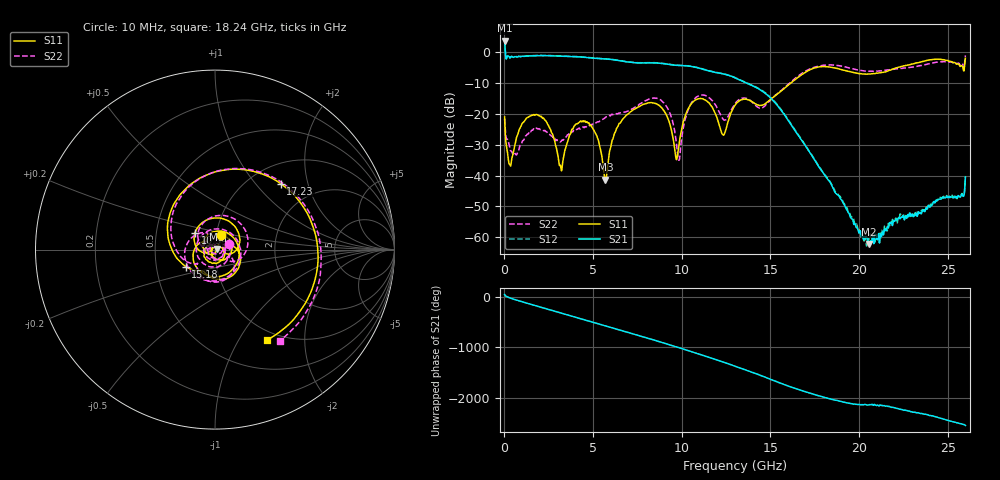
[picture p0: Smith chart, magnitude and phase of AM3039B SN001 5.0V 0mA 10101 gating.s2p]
!Agilent Technologies,E8364B,MY43040894,A.07.50.67
!Agilent E8364B: A.07.50.67
!Date: Tuesday, June 28, 2016 08:09:14
!Correction: S11(Full 2 Port(1,2))
!S21(Full 2 Port(1,2))
!S12(Full 2 Port(1,2))
!S22(Full 2 Port(1,2))
!S2P File: Measurements: S11, S21, S12, S22:
# Hz S  dB  R 50
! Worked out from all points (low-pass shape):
!   1601 points, 10 MHz to 26 GHz, reference 50 ohm
!   highest |S21| = 3.74 dB at 10 MHz (marker M1); lowest = -62.1 dB at 20.57 GHz (marker M2)
!   |S21| within 3 dB of the highest: start of sweep to 44.01 MHz
!   lowest |S11| = -41.3 dB at 5.695 GHz (marker M3), VSWR 1.02, Z = 50.9 + j0.0578 ohm
!   |S11| at or under -10 dB: start of sweep to 16.15 GHz
!   |S22| runs from -35.0 to -1.1 dB; largest |S21 - S12| = 0.025
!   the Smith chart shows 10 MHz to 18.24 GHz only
!   S11 on the Smith chart (normalised r, x): 10 MHz: 1.05, +0.18; 10.54 GHz: 0.79, +0.15; 15.18 GHz: 0.71, -0.14; 17.23 GHz: 1.36, +1.37; 18.24 GHz: 0.87, -1.33
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1e7  -20.97 68.1  3.74 40.9  3.81 41.8  -21.66 20.3
7.409688e8  -26.77 125.0  -1.51 -74.4  -1.46 -74.2  -32.56 179.9
1.69935e9  -20.40 28.8  -1.14 -172.8  -1.11 -172.6  -24.74 16.6
2.755194e9  -27.28 -101.1  -1.19 81.3  -1.12 81.5  -27.99 -159.7
3.551138e9  -29.23 21.2  -1.35 1.9  -1.28 2.0  -26.81 27.3
4.347081e9  -22.47 -91.2  -1.57 -78.8  -1.53 -78.7  -24.45 -116.6
5.695312e9  -41.34 3.8  -2.20 144.2  -2.15 144.4  -21.13 -19.6
7.076031e9  -19.50 78.0  -3.26 2.9  -3.21 3.1  -18.77 89.2
8.684162e9  -17.08 -142.4  -3.52 -162.7  -3.45 -162.6  -15.15 -159.7
9.821225e9  -31.10 -162.5  -4.28 75.6  -4.22 75.6  -34.92 124.7
1.053595e10  -16.76 140.5  -4.60 -4.3  -4.55 -4.3  -16.52 124.4
1.194916e10  -20.57 -13.8  -6.61 -164.4  -6.55 -164.5  -17.55 -28.8
1.3005e10  -17.18 -9.0  -8.29 68.4  -8.21 68.9  -16.66 -43.1
1.518166e10  -14.48 -150.0  -15.83 145.8  -15.60 146.8  -14.47 -165.4
1.722838e10  -5.70 45.1  -32.51 -103.8  -32.29 -104.2  -5.42 39.8
1.734208e10  -5.40 33.4  -33.50 -116.0  -33.36 -116.3  -5.15 29.3
1.823549e10  -4.73 -60.2  -41.17 157.5  -40.94 156.0  -4.11 -54.5
2.057459e10  -7.05 102.4  -62.11 27.0  -60.20 34.9  -6.18 113.5
2.167916e10  -5.96 26.0  -56.47 -3.2  -55.79 -15.4  -5.74 33.5
2.323856e10  -3.50 -92.1  -52.41 -131.5  -52.34 -126.0  -4.62 -80.8
2.435938e10  -2.26 176.6  -47.90 145.2  -48.36 146.2  -3.26 -166.7
2.6e10  -1.94 -11.4  -40.47 -20.7  -40.12 -20.9  -1.06 21.3
